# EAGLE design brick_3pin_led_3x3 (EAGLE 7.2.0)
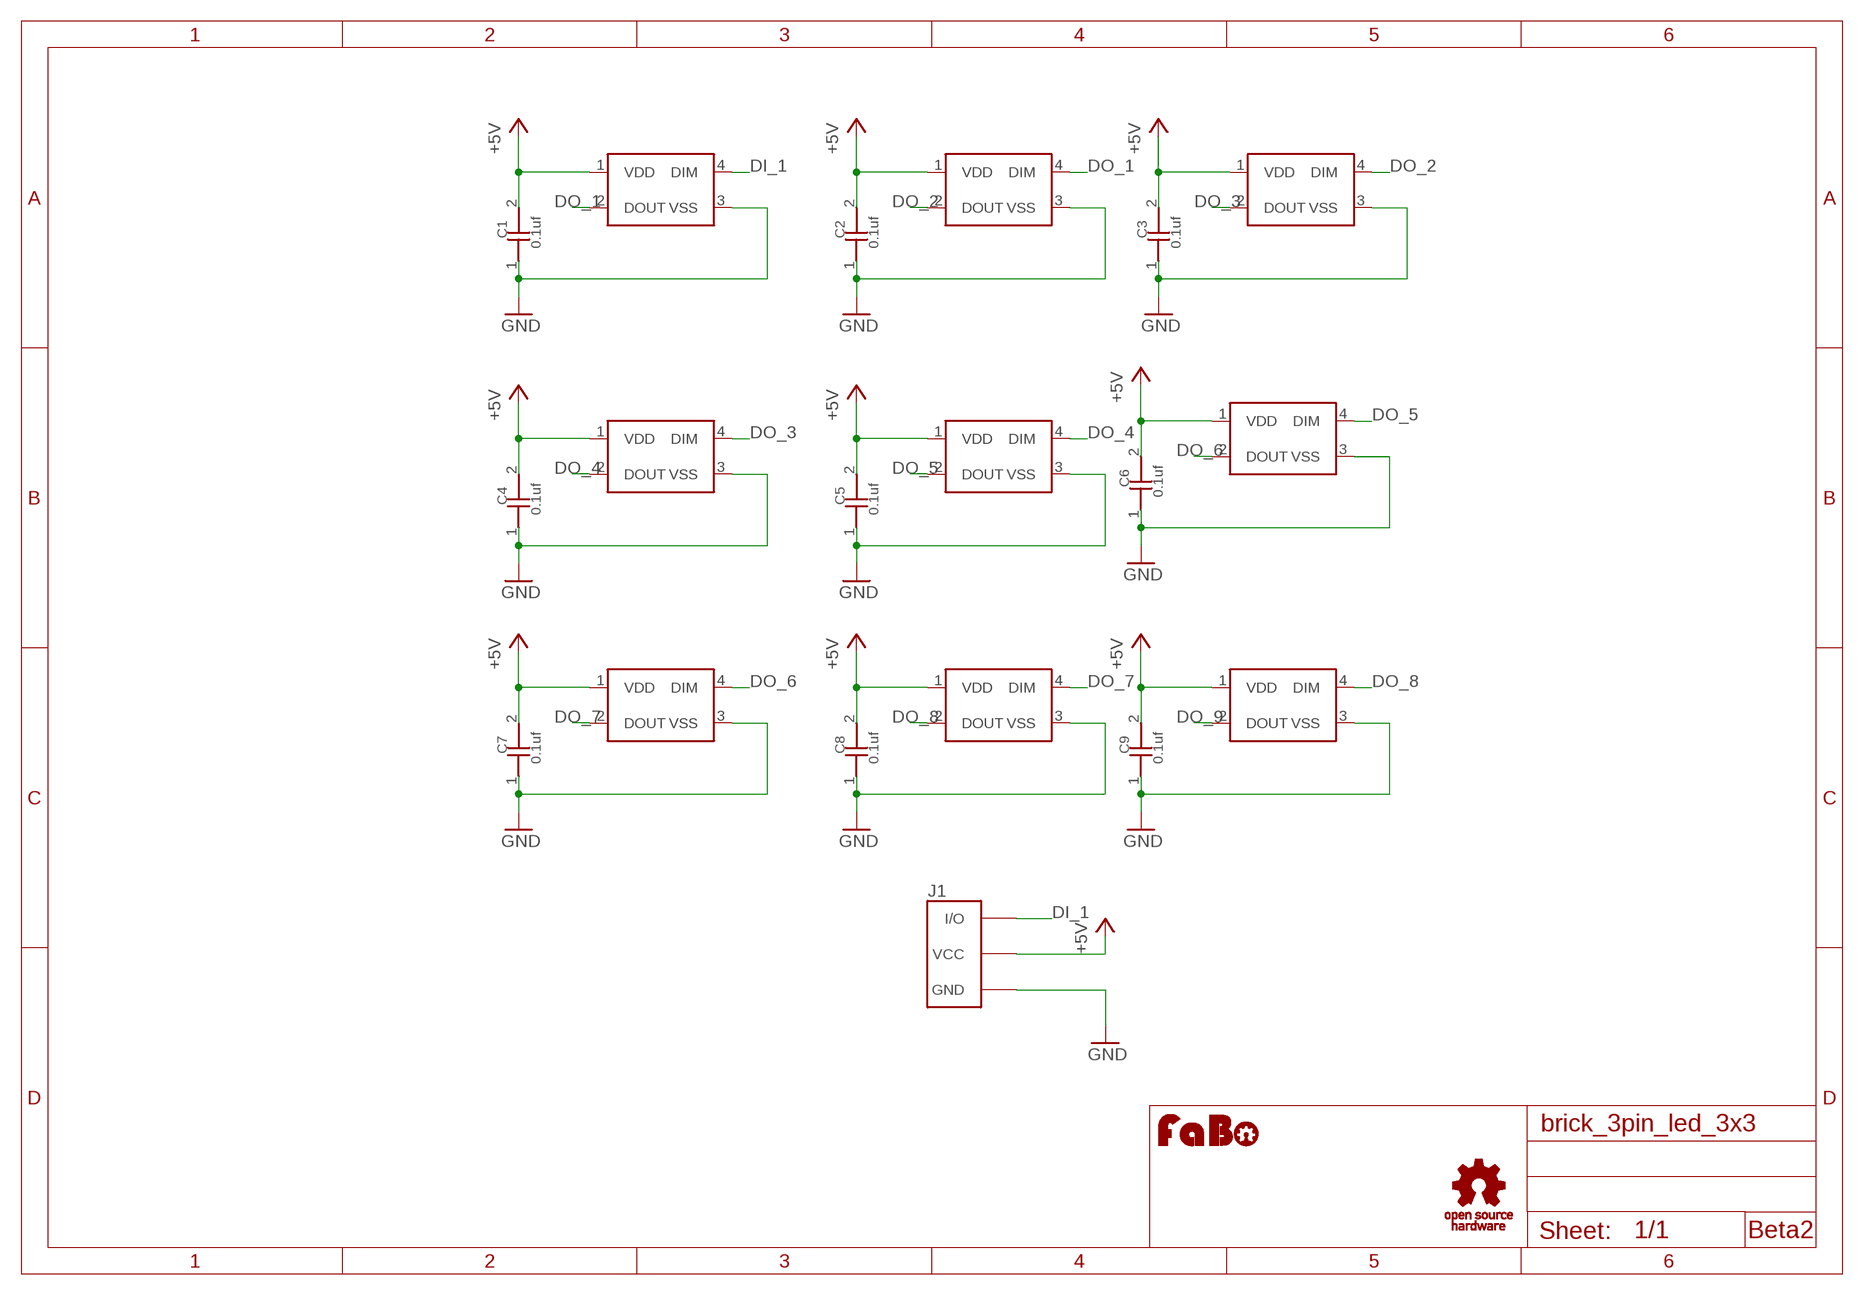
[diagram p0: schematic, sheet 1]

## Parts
C1  0.1uf  CAPACITOR0603  [0603]
C2  0.1uf  CAPACITOR0603  [0603]
C3  0.1uf  CAPACITOR0603  [0603]
C4  0.1uf  CAPACITOR0603  [0603]
C5  0.1uf  CAPACITOR0603  [0603]
C6  0.1uf  CAPACITOR0603  [0603]
C7  0.1uf  CAPACITOR0603  [0603]
C8  0.1uf  CAPACITOR0603  [0603]
C9  0.1uf  CAPACITOR0603  [0603]
J1  BRICK_3PIN_BIG  [BRICK_3PIN_BIG]
LED1  WS2818B  [WS2818B]
LED2  WS2818B  [WS2818B]
LED3  WS2818B  [WS2818B]
LED4  WS2818B  [WS2818B]
LED5  WS2818B  [WS2818B]
LED6  WS2818B  [WS2818B]
LED7  WS2818B  [WS2818B]
LED8  WS2818B  [WS2818B]
LED9  WS2818B  [WS2818B]
U$4  LOGO_OSHW_T-M  [LOGO_OSHW_T_M]
U$5  LOGO_FABO-M  [LOGO_FABO_M]

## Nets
+5V: C1.2 C2.2 C3.2 C4.2 C5.2 C6.2 C7.2 C8.2 C9.2 J1.VCC LED1.1(VDD) LED2.1(VDD) LED3.1(VDD) LED4.1(VDD) LED5.1(VDD) LED6.1(VDD) LED7.1(VDD) LED8.1(VDD) LED9.1(VDD)
DI_1: J1.IN/OUT(I/O) LED1.4(DIM)
DO_1: LED1.2(DOUT) LED2.4(DIM)
DO_2: LED2.2(DOUT) LED3.4(DIM)
DO_3: LED3.2(DOUT) LED4.4(DIM)
DO_4: LED4.2(DOUT) LED5.4(DIM)
DO_5: LED5.2(DOUT) LED6.4(DIM)
DO_6: LED6.2(DOUT) LED7.4(DIM)
DO_7: LED7.2(DOUT) LED8.4(DIM)
DO_8: LED8.2(DOUT) LED9.4(DIM)
DO_9: LED9.2(DOUT)
GND: C1.1 C2.1 C3.1 C4.1 C5.1 C6.1 C7.1 C8.1 C9.1 J1.GND LED1.3(VSS) LED2.3(VSS) LED3.3(VSS) LED4.3(VSS) LED5.3(VSS) LED6.3(VSS) LED7.3(VSS) LED8.3(VSS) LED9.3(VSS)

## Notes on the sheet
- Beta2

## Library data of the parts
C1-C9 = GClue-Capacitor:CAPACITOR
J1 = GClue:BRICK_3PIN: FaBo Brick 3pin
LED1-LED9 = GClue-LED:WS2818B
U$4 = GClue:LOGO_OSHW_T
U$5 = FaBo:LOGO_FABO

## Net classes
0 default: width 0.254 mm

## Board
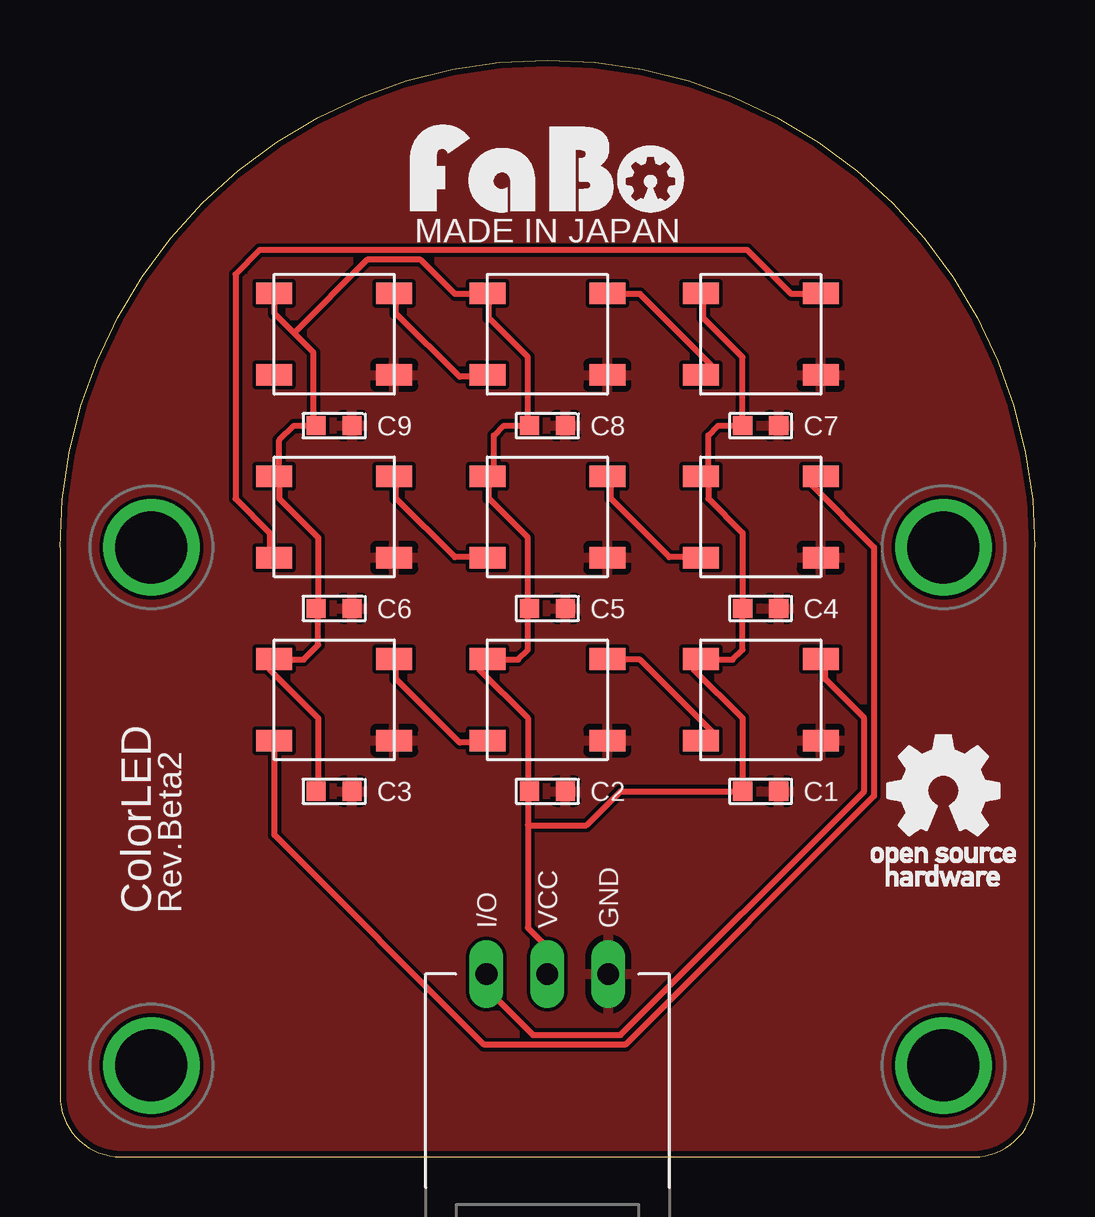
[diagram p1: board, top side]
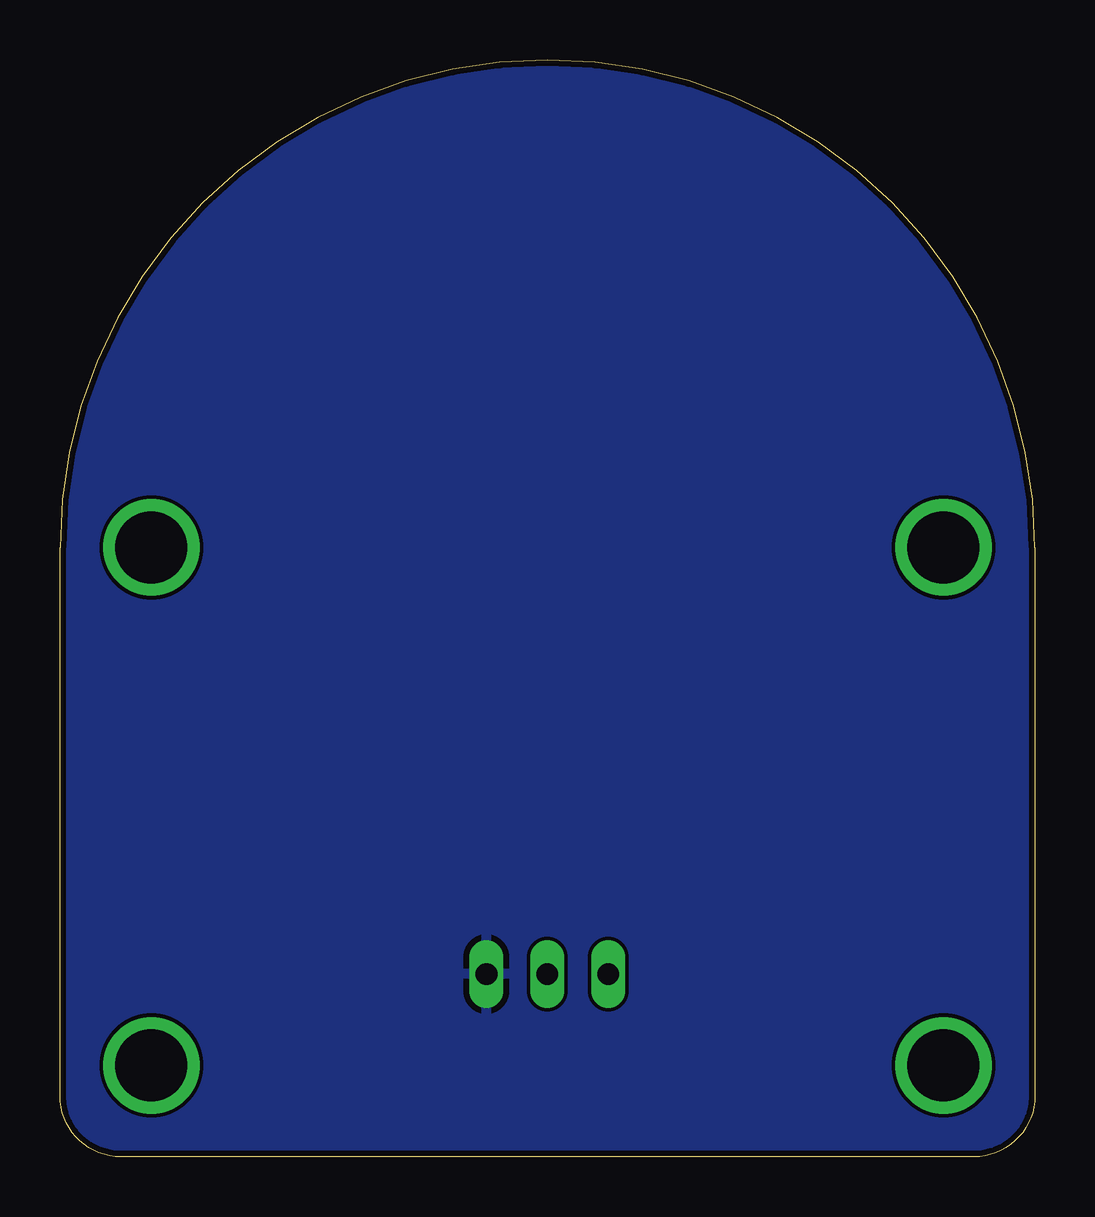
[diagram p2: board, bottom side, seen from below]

Size 40.64 x 45.72 mm. Coordinates in mm from the lower left corner, seen from the top.
Copper layers (1*16): Top 0.035mm / dielectric 1.5mm / Bottom 0.035mm
Design rules "Elecrow_2-layer_eagle_rule": minimum track width 6mil, minimum drill 12mil, track to track 6mil, track to pad 6mil, pad to pad 6mil, via to via 6mil, smd to smd 0mil, copper to edge 10mil, drill to drill 10mil, minimum pad ring 10mil, minimum via ring 6mil, stop-mask expansion 2mil, vias tented up to drill 100mil, thermal gap 10mil

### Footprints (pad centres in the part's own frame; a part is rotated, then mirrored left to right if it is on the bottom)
0603 = smd 0.8 x 0.8: 1 -0.75,0; 2 0.75,0
BRICK_3PIN_BIG = drill 0.9 long: GND 2.54,-8.89; IN/OUT -2.54,-8.89; VCC 0,-8.89 | drill 3 pad 3.81: P$5 -16.51,8.89; P$6 16.51,8.89; P$7 -16.51,-12.7; P$8 16.51,-12.7
WS2818B = smd 1.5 x 0.9: 1 -2.5,1.7; 2 -2.5,-1.7; 3 2.5,-1.7; 4 2.5,1.7

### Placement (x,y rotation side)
C1  29.21,15.24 180 top
C2  20.32,15.24 180 top
C3  11.43,15.24 180 top
C4  29.21,22.86 180 top
C5  20.32,22.86 180 top
C6  11.43,22.86 180 top
C7  29.21,30.48 180 top
C8  20.32,30.48 180 top
C9  11.43,30.48 180 top
J1  20.32,16.51 0 top
LED1  29.21,19.05 0 top
LED2  20.32,19.05 0 top
LED3  11.43,19.05 0 top
LED4  29.21,26.67 0 top
LED5  20.32,26.67 0 top
LED6  11.43,26.67 0 top
LED7  29.21,34.29 0 top
LED8  20.32,34.29 0 top
LED9  11.43,34.29 0 top
U$4  36.83,15.24 0 top
U$5  20.32,39.37 0 top

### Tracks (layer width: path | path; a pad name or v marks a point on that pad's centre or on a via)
+5V
  Top 0.254: 28.45,15.24 28.45,18.29 26.42,20.32 26.42,20.52 26.62,20.73 LED1.1 26.82,20.73 28.04,20.73 28.45,21.13 28.45,22.76 C4.2 28.45,22.96 28.45,26.01 27.03,27.43 27.03,28.65 | 28.45,30.48 27.43,30.48 27.03,30.07 27.03,28.65 | 27.03,28.65 26.82,28.45 LED4.1 27.03,28.65 | 28.45,30.48 28.45,33.33 26.82,34.95 26.82,35.97 LED7.1 | 28.45,30.48 C7.2 | C3.2 10.77,15.24 10.77,18.29 8.74,20.32 8.74,20.73 LED3.1 8.94,20.73 10.16,20.73 10.77,21.34 10.77,22.76 C6.2 10.77,22.96 10.77,25.81 9.14,27.43 9.14,28.65 | 10.57,30.48 9.75,30.48 9.14,29.87 9.14,28.65 | 9.14,28.65 8.94,28.45 LED6.1 9.14,28.65 | 9.75,34.34 10.57,33.53 10.57,30.48 | 9.75,34.34 8.94,35.15 8.94,35.97 LED9.1 | 10.57,30.48 C9.2 | 19.51,30.48 18.49,30.48 18.09,30.07 18.09,28.65 17.88,28.45 LED5.1 17.88,28.25 17.88,27.43 19.51,25.81 19.51,22.96 C5.2 19.51,22.76 19.51,21.13 19.1,20.73 17.88,20.73 LED2.1 17.68,20.73 17.48,20.52 17.48,20.32 19.51,18.29 19.51,15.24 | 19.51,30.48 19.51,33.33 17.88,34.95 17.88,35.97 LED8.1 17.68,35.97 16.46,35.97 15.04,37.39 12.8,37.39 9.75,34.34 | 19.51,30.48 C8.2 | J1.VCC 20.32,8.74 19.51,9.55 19.51,13.82 | 19.51,15.24 19.51,13.82 | 19.51,15.24 C2.2 | 28.45,15.24 23.37,15.24 21.95,13.82 19.51,13.82 | 28.45,15.24 C1.2
DI_1
  Top 0.254: LED1.4 31.9,20.73 31.9,19.91 33.53,18.29 33.53,15.24 23.37,5.08 19.71,5.08 17.88,6.91 17.88,7.52 J1.IN/OUT
DO_1
  Top 0.254: LED2.4 22.96,20.73 24.18,20.73 27.23,17.68 26.82,17.27 LED1.2
DO_2
  Top 0.254: LED3.4 14.02,20.73 14.02,19.91 16.66,17.27 17.68,17.27 LED2.2
DO_3
  Top 0.254: LED3.2 8.94,17.27 8.94,13.41 17.68,4.67 23.57,4.67 33.93,15.04 33.93,25.4 31.29,28.04 31.7,28.45 LED4.4
DO_4
  Top 0.254: LED5.4 22.96,28.25 22.96,27.43 25.4,24.99 26.62,24.99 LED4.2
DO_5
  Top 0.254: LED6.4 14.02,28.25 14.02,27.43 16.46,24.99 17.68,24.99 LED5.2
DO_6
  Top 0.254: LED6.2 8.74,24.99 8.74,26.01 7.32,27.43 7.32,36.78 8.33,37.8 28.65,37.8 30.48,35.97 31.7,35.97 LED7.4
DO_7
  Top 0.254: LED8.4 22.96,35.97 24.18,35.97 27.23,32.92 26.82,32.51 LED7.2
DO_8
  Top 0.254: LED9.4 14.02,35.97 14.02,35.15 16.66,32.51 17.68,32.51 LED8.2
GND
  pour Bottom: -1.27,-1.27 41.91,-1.27 41.91,46.99 -1.27,46.99
  pour Top: -1.27,-1.27 41.91,-1.27 41.91,46.99 -1.27,46.99

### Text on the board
tPlace: MADE IN JAPAN | ColorLED | Rev.Beta2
